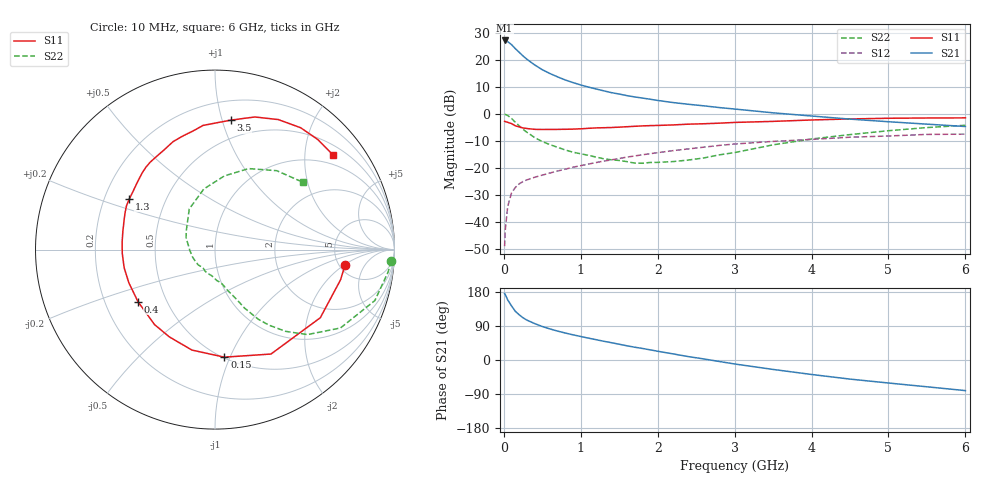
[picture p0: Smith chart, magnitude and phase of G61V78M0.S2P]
! SIEMENS Small Signal Semiconductors
! BFG193
! Si NPN RF Bipolar Junction Transistor in SOT223
! VCE = 1.75 V  IC = 8 mA
! Common Emitter S-Parameters:  August  1996
# GHz  S  MA  R  50
!  f  S11  S21  S12  S22
! GHz  MAG  ANG  MAG  ANG  MAG  ANG  MAG  ANG
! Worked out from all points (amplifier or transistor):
!   36 points, 10 MHz to 6 GHz, reference 50 ohm
!   highest |S21| = 27.1 dB at 10 MHz (marker M1)
!   |S21| within 3 dB of that: start of sweep to 148.6 MHz
!   unconditionally stable (mu >= 1): 926.2 MHz to 2.777 GHz
!   at 250 MHz: K = 0.47, MSG = 23.2 dB, |S12| = -25.0 dB
!   at 1.4 GHz: K = 1.08, MAG = 10.7 dB, |S12| = -17.0 dB
!   at 6 GHz: K = 0.92, MSG = 1.4 dB, |S12| = -7.5 dB
!   S11 on the Smith chart (normalised r, x): 10 MHz: 5.61, -2.07; 150 MHz: 0.51, -0.95; 400 MHz: 0.34, -0.27; 1.3 GHz: 0.31, +0.25; 3.5 GHz: 0.35, +1.07; 6 GHz: 0.74, +2.68
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0.01  0.7294 -6.8  22.7 175.4  0.0036 91.6  0.9831 -3.7
0.02  0.7196 -13.5  22.59 172.0  0.0075 85.4  0.9729 -7.3
0.05  0.6988 -32.9  21.62 158.7  0.0194 74.0  0.9348 -17.7
0.1  0.6602 -61.8  18.99 142.7  0.0347 63.8  0.8241 -32.0
0.15  0.6016 -85.0  15.99 128.4  0.0438 54.5  0.6995 -42.6
0.2  0.5744 -102.9  13.7 119.2  0.051 50.3  0.6016 -49.2
0.25  0.549 -117.5  11.72 111.3  0.0564 46.8  0.5167 -54.5
0.3  0.5367 -128.9  10.2 105.2  0.0604 45.6  0.4574 -58.1
0.4  0.5179 -146.0  8.032 96.2  0.0674 44.2  0.3653 -63.2
0.5  0.5144 -159.1  6.539 88.3  0.0739 43.4  0.3075 -66.2
0.6  0.516 -168.6  5.555 82.0  0.0809 43.8  0.2699 -69.2
0.7  0.5171 -177.5  4.816 76.2  0.088 44.5  0.2409 -72.5
0.9  0.5231 168.9  3.78 66.4  0.1034 44.2  0.1957 -78.1
1.1  0.5408 158.1  3.122 57.7  0.1184 43.6  0.1716 -87.0
1.3  0.555 149.2  2.662 49.4  0.1343 42.1  0.1478 -96.2
1.7  0.5891 133.5  2.056 33.8  0.1668 37.5  0.1232 -122.0
2.2  0.6247 116.7  1.618 16.1  0.2093 28.9  0.1315 -160.7
2.8  0.6732 100.2  1.308 -3.9  0.2613 17.3  0.1749 157.3
3.5  0.7264 83.1  1.046 -24.9  0.3102 1.2  0.2681 122.3
4.5  0.8059 64.0  0.8 -50.4  0.3705 -18.4  0.4141 82.7
5.5  0.8391 47.0  0.646 -70.7  0.4174 -42.1  0.5585 51.9
6  0.8434 38.5  0.584 -80.8  0.4216 -55.7  0.6159 37.6
